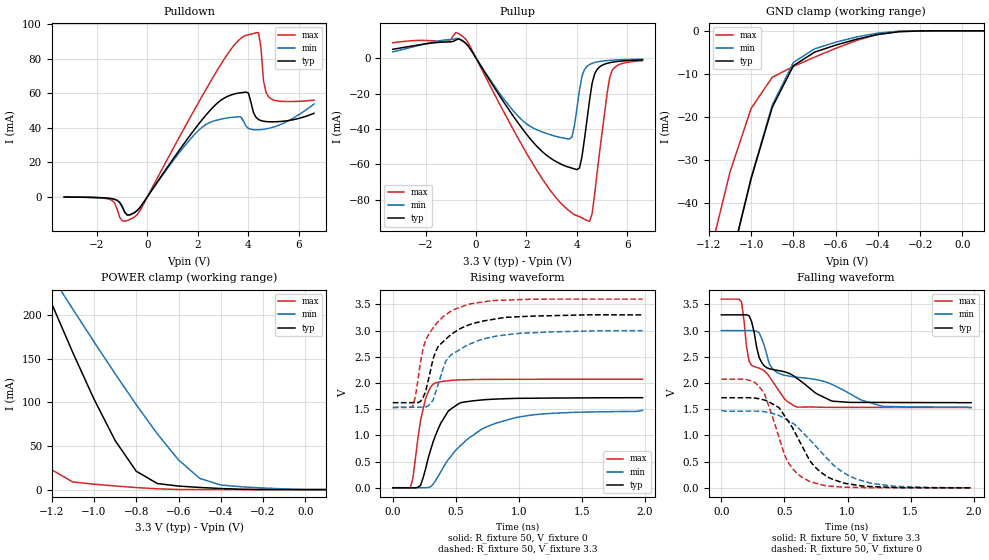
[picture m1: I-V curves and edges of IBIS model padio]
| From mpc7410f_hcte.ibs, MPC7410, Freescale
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| *   padio Model   *
[Model]   padio
Model_type   I/O
Polarity   Non-Inverting
Vinl = 0.8V
Vinh = 2V
Vmeas = 1.65V
Cref = 0
Rref = 50
Vref = 1.65V
|   typ   min   max
C_comp   2.091940e-12   1.793850e-12   2.185370e-12
|   typ   min   max
[Voltage range]   3.3V   3.0V   3.6V
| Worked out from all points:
|   slope of the pulldown table from 0 to 0.495 V, typ, clamps not added: 45.9 ohm
|   slope of the pullup table from 0 to 0.495 V, typ, clamps not added: 43.2 ohm
|   GND clamp passes 1 mA (typ) near -0.41 V on its own axis
|   POWER clamp passes 1 mA (typ) near -0.37 V on its own axis
|   falling waveform, R_fixture 50, V_fixture 3.3: 20-80 % time 410ps typ, 656ps min, 250ps max; typ from 3.3 V to 1.63 V
|   rising waveform, R_fixture 50, V_fixture 0: 20-80 % time 159ps typ, 384ps min, 84.1ps max; typ from 0.002 V to 1.72 V
|   falling waveform, R_fixture 50, V_fixture 0: 20-80 % time 265ps typ, 372ps min, 188ps max; typ from 1.72 V to 0.003 V
|   rising waveform, R_fixture 50, V_fixture 3.3: 20-80 % time 214ps typ, 238ps min, 174ps max; typ from 1.62 V to 3.3 V
[Pulldown]
|   Voltage   I(typ)   I(min)   I(max)
-3.3V     -216.8uA   -217uA     -234uA
-1.5V     -979.3uA   -969uA     -1.583mA
-1V       -5.813mA   -5.602mA   -13.94mA
-400mV    -7.939mA   -7.955mA   -10.3mA
2.2V      45.21mA    40.66mA    59.15mA
3.6V      60.07mA    46.33mA    90.52mA
3.9V      60.68mA    41.01mA    93.61mA
4.4V      44.79mA    38.83mA    95.19mA
4.5V      44.13mA    38.93mA    86.25mA
4.6V      43.77mA    39.1mA     67.23mA
4.8V      43.47mA    39.62mA    57.95mA
6.6V      48.37mA    53.7mA     55.97mA
[GND_clamp]
-3.3V     -642.8mA   -642.9mA   -621.3mA
-1.2V     -76.69mA   -76.65mA   -52.95mA
-1.1V     -54.53mA   -54.43mA   -32.86mA
-1V       -34.4mA    -34.17mA   -18.04mA
-900mV    -17.77mA   -17.28mA   -10.81mA
-800mV    -8.12mA    -7.356mA   -8.277mA
-700mV    -4.964mA   -4.197mA   -6.127mA
-600mV    -3.326mA   -2.657mA   -4.085mA
-500mV    -1.945mA   -1.416mA   -2.228mA
-400mV    -853.1uA   -525.7uA   -766.9uA
-300mV    -220.3uA   -102.6uA   -84.07uA
100mV     0A         0A         0A
[Pullup]
-3.3V     4.946mA    3.465mA    8.64mA
-500mV    9.355mA    9.474mA    11.91mA
1.8V      -39.18mA   -34.71mA   -48.63mA
3.7V      -61.68mA   -45.73mA   -86.31mA
3.9V      -62.57mA   -38.16mA   -88.39mA
4.1V      -62.03mA   -18.09mA   -89.51mA
4.3V      -45.46mA   -6.466mA   -90.95mA
4.5V      -23.8mA    -3.627mA   -92.13mA
4.7V      -8.941mA   -2.511mA   -76.99mA
5.3V      -2.616mA   -1.3mA     -10.79mA
5.6V      -1.935mA   -1.046mA   -4.176mA
6.6V      -1.035mA   -635.5uA   -1.486mA
[POWER_clamp]
-3.3V     1.509A     1.073A     1.768A
-1.5V     390.6mA    360.8mA    223.6mA
-1.3V     271.5mA    283.4mA    74.83mA
-1.2V     213.5mA    245.1mA    22.75mA
-1.1V     157.2mA    207.2mA    8.729mA
-900mV    56.41mA    133.1mA    4.171mA
-800mV    21.12mA    97.5mA     2.348mA
-700mV    6.964mA    63.89mA    902.3uA
-600mV    4.047mA    34.11mA    147.7uA
-500mV    2.488mA    12.92mA    7.953uA
-400mV    1.246mA    5.256mA    2.334uA
100mV     0A         0A         0A
|   typ   min   max
[Ramp]
dV/dt_r   1.03065/1.58970e-10   0.87515/3.71954e-10   1.24306/8.33383e-11
dV/dt_f   1.00534/4.10800e-10   0.87700/6.52613e-10   1.24008/2.50211e-10
[Falling Waveform]
R_fixture = 50
V_fixture = 3.3
V_fixture_min = 3.0
V_fixture_max = 3.6
| time   V(typ)   V(min)   V(max)
0s        3.3V       3V         3.6V
160ps     3.3V       3V         3.545V
200ps     3.3V       3V         2.678V
220ps     3.284V     3V         2.412V
320ps     2.39V      2.845V     2.263V
400ps     2.262V     2.289V     2.054V
580ps     2.125V     2.115V     1.561V
880ps     1.655V     1.971V     1.537V
1.28ns    1.63V      1.555V     1.535V
1.98ns    1.626V     1.532V     1.534V
[Rising Waveform]
R_fixture = 50
V_fixture = 0
V_fixture_min = 0
V_fixture_max = 0
| time   V(typ)   V(min)   V(max)
0s        1.753mV    1.862mV    1.229mV
140ps     1.385mV    1.745mV    7.884mV
160ps     613.3uV    1.718mV    192.1mV
220ps     45.57mV    802.8uV    1.281V
260ps     360.7mV    1.551mV    1.7V
340ps     1.008V     142.8mV    2.001V
440ps     1.464V     536.8mV    2.043V
520ps     1.6V       766.5mV    2.057V
820ps     1.693V     1.234V     2.068V
1.98ns    1.719V     1.477V     2.073V
[Falling Waveform]
R_fixture = 50
V_fixture = 0
V_fixture_min = 0
V_fixture_max = 0
| time   V(typ)   V(min)   V(max)
0s        1.72V      1.477V     2.073V
220ps     1.72V      1.465V     2.053V
320ps     1.689V     1.46V      1.871V
340ps     1.676V     1.454V     1.81V
460ps     1.523V     1.379V     941.9mV
520ps     1.308V     1.297V     528.2mV
700ps     523.9mV    921.3mV    121.8mV
860ps     188mV      506.4mV    34.74mV
1.1ns     43.54mV    147.5mV    7.842mV
1.98ns    2.542mV    3.89mV     1.572mV
[Rising Waveform]
R_fixture = 50
V_fixture = 3.3
V_fixture_min = 3.0
V_fixture_max = 3.6
| time   V(typ)   V(min)   V(max)
0s        1.624V     1.532V     1.533V
160ps     1.624V     1.538V     1.561V
220ps     1.649V     1.538V     2.399V
260ps     1.83V      1.542V     2.808V
320ps     2.464V     1.676V     3.051V
360ps     2.697V     1.973V     3.17V
420ps     2.834V     2.413V     3.305V
500ps     2.986V     2.591V     3.415V
940ps     3.256V     2.931V     3.584V
1.98ns    3.299V     2.998V     3.599V
